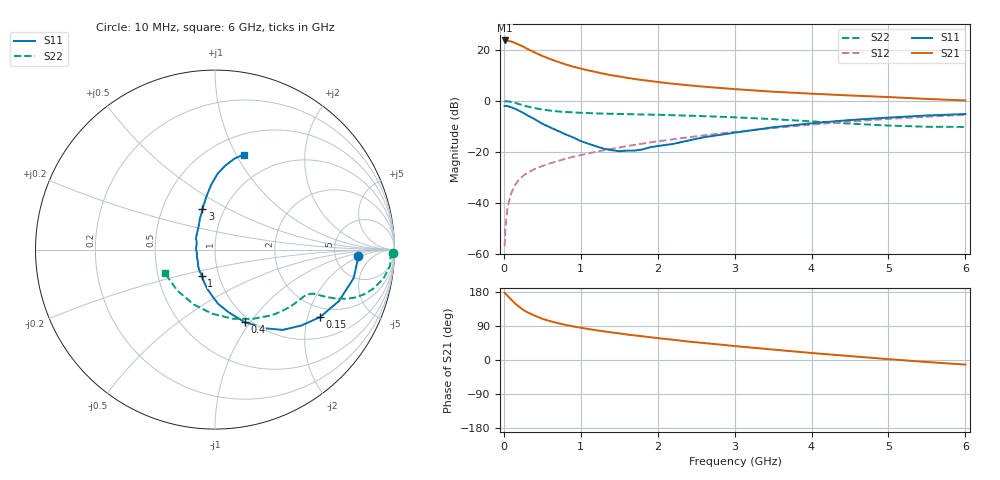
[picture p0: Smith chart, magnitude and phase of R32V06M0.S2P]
! SIEMENS Small Signal Semiconductors
! BFR181
! Si NPN RF Bipolar Junction Transistor in SOT23
! VCE = 2 V  IC = 6 mA
! Common Emitter S-Parameters:  May  1996
# GHz  S  MA  R  50
!  f  S11  S21  S12  S22
! GHz  MAG  ANG  MAG  ANG  MAG  ANG  MAG  ANG
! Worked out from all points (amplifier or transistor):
!   36 points, 10 MHz to 6 GHz, reference 50 ohm
!   highest |S21| = 23.8 dB at 10 MHz (marker M1)
!   |S21| within 3 dB of that: start of sweep to 287.7 MHz
!   unconditionally stable (mu >= 1): 957.6 MHz to 2.846 GHz
!   at 250 MHz: K = 0.47, MSG = 25.4 dB, |S12| = -29.5 dB
!   at 1.4 GHz: K = 1.06, MAG = 12.9 dB, |S12| = -18.8 dB
!   at 6 GHz: K = 0.86, MSG = 2.8 dB, |S12| = -5.5 dB
!   S11 on the Smith chart (normalised r, x): 10 MHz: 8.54, -1.63; 150 MHz: 1.65, -2.40; 400 MHz: 0.94, -0.94; 1 GHz: 0.83, -0.25; 3 GHz: 0.79, +0.38; 6 GHz: 0.70, +1.07
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0.01  0.7971 -2.5  15.41 177.7  0.0014 87.4  0.9897 -1.0
0.02  0.7964 -4.5  15.35 175.3  0.0032 88.5  0.9792 -2.1
0.05  0.7889 -11.6  15.18 169.0  0.0085 85.3  0.9794 -5.2
0.1  0.7478 -22.5  14.65 158.7  0.0159 79.2  0.9521 -9.8
0.15  0.6958 -32.7  13.65 148.4  0.0228 73.6  0.9079 -13.9
0.2  0.6408 -41.3  12.68 140.3  0.0289 70.2  0.8655 -16.8
0.25  0.5856 -49.8  11.69 132.6  0.0336 68.2  0.8219 -19.0
0.3  0.526 -56.7  10.67 126.5  0.0381 66.7  0.7825 -20.5
0.4  0.4381 -67.7  8.985 117.3  0.0459 64.4  0.7228 -22.1
0.5  0.3569 -77.8  7.638 108.8  0.0526 63.9  0.6783 -23.0
0.6  0.3031 -86.6  6.661 102.6  0.0593 64.1  0.6453 -23.4
0.8  0.2212 -101.5  5.231 92.7  0.0725 64.7  0.606 -24.0
1  0.1627 -117.2  4.313 85.0  0.0862 65.6  0.5844 -25.0
1.1  0.1438 -127.6  3.978 81.8  0.0932 65.8  0.5763 -25.7
1.3  0.1151 -146.2  3.414 75.7  0.1075 65.8  0.5632 -27.1
1.6  0.1055 179.3  2.842 67.3  0.1294 65.5  0.5501 -30.0
2.2  0.1428 132.8  2.169 53.4  0.1765 63.5  0.5242 -37.6
3  0.2375 107.1  1.706 36.8  0.2458 58.3  0.4762 -50.8
3.5  0.303 98.9  1.517 27.5  0.2928 54.2  0.4384 -61.8
4.5  0.4212 88.2  1.279 10.3  0.3926 43.4  0.3576 -92.4
5.5  0.517 78.1  1.094 -5.3  0.4893 30.4  0.3101 -132.8
6  0.5533 73.2  1.021 -12.1  0.5323 23.3  0.3084 -154.6
